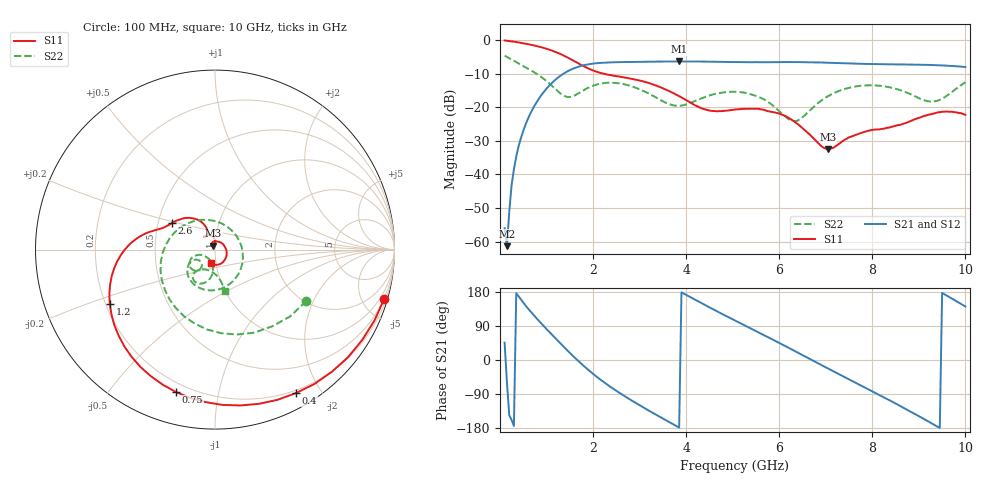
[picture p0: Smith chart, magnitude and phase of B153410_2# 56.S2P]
!  2-Port S-parameters saved by WinCal
! VAR MeasName=S-Parameters (CALIBRATED_DATA) read from VNA (N5245A)
! VAR MeasDate=2016-12-23 10:02:19
! VAR NAME=B153410_2# 56
! VAR FILENAME=B153410_2# 56.S2P
! VAR DATE=2016-12-23 10:02:19
! VAR PHYS_PORTS=1,2
# Hz S DB R 50
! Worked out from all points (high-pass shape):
!   199 points, 100 MHz to 10 GHz, reference 50 ohm
!   highest |S21| = -6.39 dB at 3.85 GHz (marker M1); lowest = -61.4 dB at 150 MHz (marker M2)
!   |S21| within 3 dB of the highest: 1.443 GHz to end of sweep
!   lowest |S11| = -32.4 dB at 7.05 GHz (marker M3), VSWR 1.05, Z = 49 + j2.13 ohm
!   |S11| at or under -10 dB: 2.212 GHz to end of sweep
!   |S22| runs from -24.2 to -4.7 dB; largest |S21 - S12| = 0.0024
!   S11 on the Smith chart (normalised r, x): 100 MHz: 0.45, -6.99; 400 MHz: 0.17, -1.70; 750 MHz: 0.15, -0.75; 1.2 GHz: 0.22, -0.23; 2.6 GHz: 0.59, +0.19; 10 GHz: 0.95, -0.14
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1e8  -0.16 -16.2  -56.01 45.8  -58.78 5.4  -4.67 -29.4
1.5e8  -0.24 -23.9  -61.36 -58.4  -60.61 -131.4  -5.04 -41.8
2.5e8  -0.41 -39.0  -43.14 -158.2  -43.25 -158.2  -5.82 -64.7
4e8  -0.74 -60.5  -31.64 168.2  -31.61 168.4  -6.99 -95.8
7.5e8  -1.69 -105.4  -19.37 115.0  -19.37 115.3  -9.74 -158.5
1.2e9  -3.60 -152.6  -11.73 56.1  -11.69 56.1  -14.75 115.2
1.45e9  -5.21 -173.2  -9.34 25.0  -9.31 24.8  -16.98 47.9
1.75e9  -7.47 169.9  -7.70 -10.2  -7.69 -10.3  -15.36 -27.1
2.2e9  -9.95 157.9  -6.79 -55.5  -6.80 -55.6  -12.92 -90.3
2.6e9  -10.98 148.4  -6.59 -89.3  -6.59 -89.4  -13.00 -124.3
3.4e9  -13.80 122.9  -6.45 -147.6  -6.45 -147.7  -17.50 -154.0
3.85e9  -16.73 112.9  -6.39 -178.3  -6.41 -178.3  -19.62 -138.8
4.5e9  -21.02 121.6  -6.48 139.0  -6.48 138.9  -16.53 -129.2
5.05e9  -20.73 129.9  -6.58 104.1  -6.60 104.1  -15.42 -143.9
5.65e9  -20.74 116.2  -6.65 66.9  -6.64 66.9  -17.51 -161.1
6.3e9  -24.02 94.1  -6.60 25.8  -6.60 25.9  -24.10 -134.2
6.7e9  -28.76 89.2  -6.64 0.1  -6.67 0.1  -20.41 -97.6
7.05e9  -32.44 114.4  -6.79 -22.5  -6.80 -22.4  -16.72 -97.2
7.7e9  -27.98 118.7  -7.06 -63.8  -7.09 -63.6  -13.73 -112.9
8.35e9  -26.09 57.2  -7.27 -105.1  -7.27 -104.9  -14.02 -128.2
9.3e9  -21.94 -50.6  -7.46 -168.9  -7.48 -168.8  -18.35 -106.8
1e10  -22.29 -105.4  -8.06 141.1  -8.07 141.3  -12.58 -76.8
